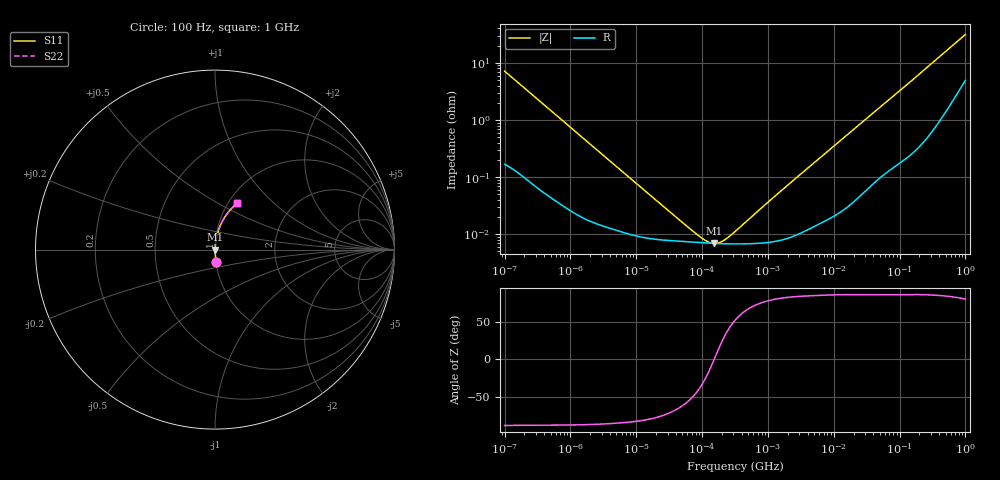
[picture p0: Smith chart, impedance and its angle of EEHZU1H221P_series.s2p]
!  *** S-Parameter ***
!  Copyright (C) Panasonic Industry
!  Conductive Polymer Hybrid Aluminum Electrolytic Capacitor
!  Parts No. EEHZU1H221P
!  Connection Mode : Series
!  1  o---||---o  2
!  GND o--------o GND
!  Conditions : Temperature = 20   DC Bias = 0 V
! Frequency Range : 100Hz  -  1GHz  [ 401 Steps ]
# Hz S RI R 50
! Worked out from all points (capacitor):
!   401 points, 100 Hz to 1 GHz, reference 50 ohm
!   read as one part in series: C = 221 uF near 108.4 Hz
!   lowest |Z| = 6.91 mohm at 153.1 kHz (marker M1)
!   series resonance near 152.5 kHz, so ESL is about 4.9 nH
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100  0.00674 -0.071  0.9933 0.071  0.9933 0.071  0.00674 -0.071
108.3927  0.00593 -0.0656  0.9941 0.0656  0.9941 0.0656  0.00593 -0.0656
296.8247  0.00128 -0.0246  0.9987 0.0246  0.9987 0.0246  0.00128 -0.0246
1487.647  0.000223 -0.00503  0.9998 0.00503  0.9998 0.00503  0.000223 -0.00503
22130.95  8.06e-05 -0.000348  0.9999 0.000348  0.9999 0.000348  8.06e-05 -0.000348
60603.82  7.39e-05 -0.000112  0.9999 0.000112  0.9999 0.000112  7.39e-05 -0.000112
80352.61  7.22e-05 -7.35e-05  0.9999 7.35e-05  0.9999 7.35e-05  7.22e-05 -7.35e-05
90677.6  7.15e-05 -5.85e-05  0.9999 5.85e-05  0.9999 5.85e-05  7.15e-05 -5.85e-05
153108.7  6.91e-05 4.63e-07  0.9999 -4.63e-07  0.9999 -4.63e-07  6.91e-05 4.63e-07
269153.5  6.79e-05 6.64e-05  0.9999 -6.64e-05  0.9999 -6.64e-05  6.79e-05 6.64e-05
291742.7  6.78e-05 7.71e-05  0.9999 -7.71e-05  0.9999 -7.71e-05  6.78e-05 7.71e-05
316227.8  6.78e-05 8.84e-05  0.9999 -8.84e-05  0.9999 -8.84e-05  6.78e-05 8.84e-05
1148154  7.35e-05 0.000411  0.9999 -0.000411  0.9999 -0.000411  7.35e-05 0.000411
4704354  0.000134 0.00167  0.9999 -0.00167  0.9999 -0.00167  0.000134 0.00167
2.357762e7  0.000499 0.00801  0.9995 -0.00801  0.9995 -0.00801  0.000499 0.00801
6.99842e7  0.00182 0.0228  0.9982 -0.0228  0.9982 -0.0228  0.00182 0.0228
1.504874e8  0.00478 0.0477  0.9952 -0.0477  0.9952 -0.0477  0.00478 0.0477
2.867477e8  0.0136 0.0892  0.9864 -0.0892  0.9864 -0.0892  0.0136 0.0892
4.120975e8  0.0259 0.1257  0.9741 -0.1257  0.9741 -0.1257  0.0259 0.1257
5.688529e8  0.0465 0.1678  0.9535 -0.1678  0.9535 -0.1678  0.0465 0.1678
8.861352e8  0.1011 0.2385  0.8989 -0.2385  0.8989 -0.2385  0.1011 0.2385
1e9  0.1234 0.2587  0.8766 -0.2587  0.8766 -0.2587  0.1234 0.2587
